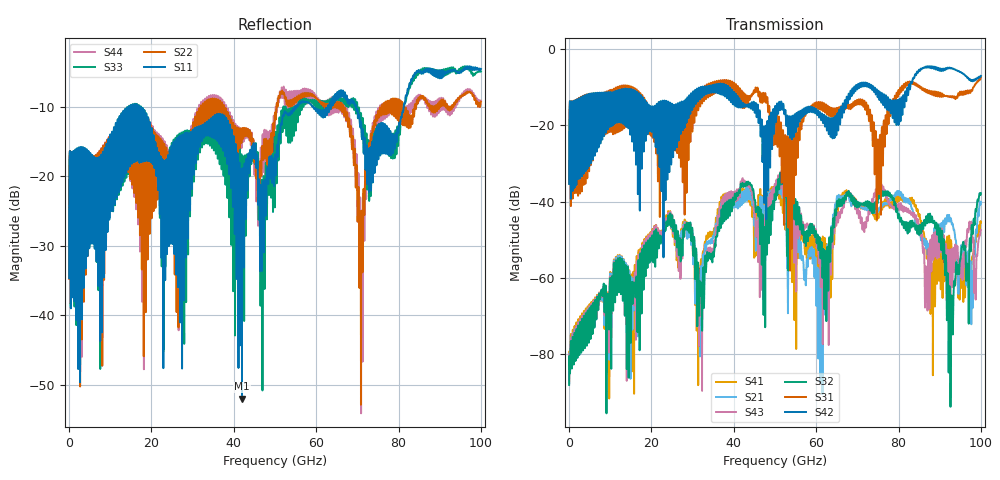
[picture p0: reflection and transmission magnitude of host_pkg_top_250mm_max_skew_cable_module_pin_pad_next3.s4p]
# Hz S RI R 50
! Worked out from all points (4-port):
!   10000 points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, 10 MHz to 100 GHz, reference 50 ohm
!   strongest paths, dB at 10 MHz, 25.01 GHz, 50.01 GHz, 75.01 GHz, 100 GHz:
!     S42: -35.3, -14.4, -15.0, -11.9, -7.0
!     S31: -35.2, -20.6, -16.6, -23.9, -7.4
!     S32: -88.1, -43.5, -38.5, -38.9, -37.8
!     S43: -87.7, -43.4, -35.5, -36.2, -47.5
!     S21: -87.5, -43.5, -37.1, -42.6, -40.1
!     S41: -87.1, -43.5, -36.7, -43.6, -45.5
!   lowest |S11| = -52.0 dB at 41.99 GHz (marker M1), VSWR 1.01, Z = 49.9 - j0.22 ohm
!   |S11| at or under -10 dB: start of sweep to 14.55 GHz; 16.92 GHz to 55.16 GHz (38.24 GHz wide, 106 % of centre); 69.67 GHz to 81.26 GHz (11.59 GHz wide, 15.4 % of centre)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
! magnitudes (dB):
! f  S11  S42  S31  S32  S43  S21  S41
! 10 MHz  -34.7  -35.3  -35.2  -88.1  -87.7  -87.5  -87.1
! 31.93 GHz  -12.7  -10.3  -12.7  -64.6  -68.7  -58.9  -56.5
! 41.99 GHz  -52.0  -15.3  -12.3  -35.8  -35.2  -38.6  -37.8
! 60.57 GHz  -10.4  -16.6  -14.0  -52.6  -54.4  -68.9  -53.9
! 77.39 GHz  -16.3  -12.6  -16.3  -37.2  -40.1  -40.3  -41.0
! 92.91 GHz  -4.7  -5.0  -12.6  -65.3  -54.0  -45.9  -53.4
! 100 GHz  -4.6  -7.0  -7.4  -37.8  -47.5  -40.1  -45.5
